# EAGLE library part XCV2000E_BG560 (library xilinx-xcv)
xcv2000e_bg560 edit this description Auto generated by make-symbol-device-package-bsdl.ulp Rev. 26 Source: xcv2000e_bg560.bsd
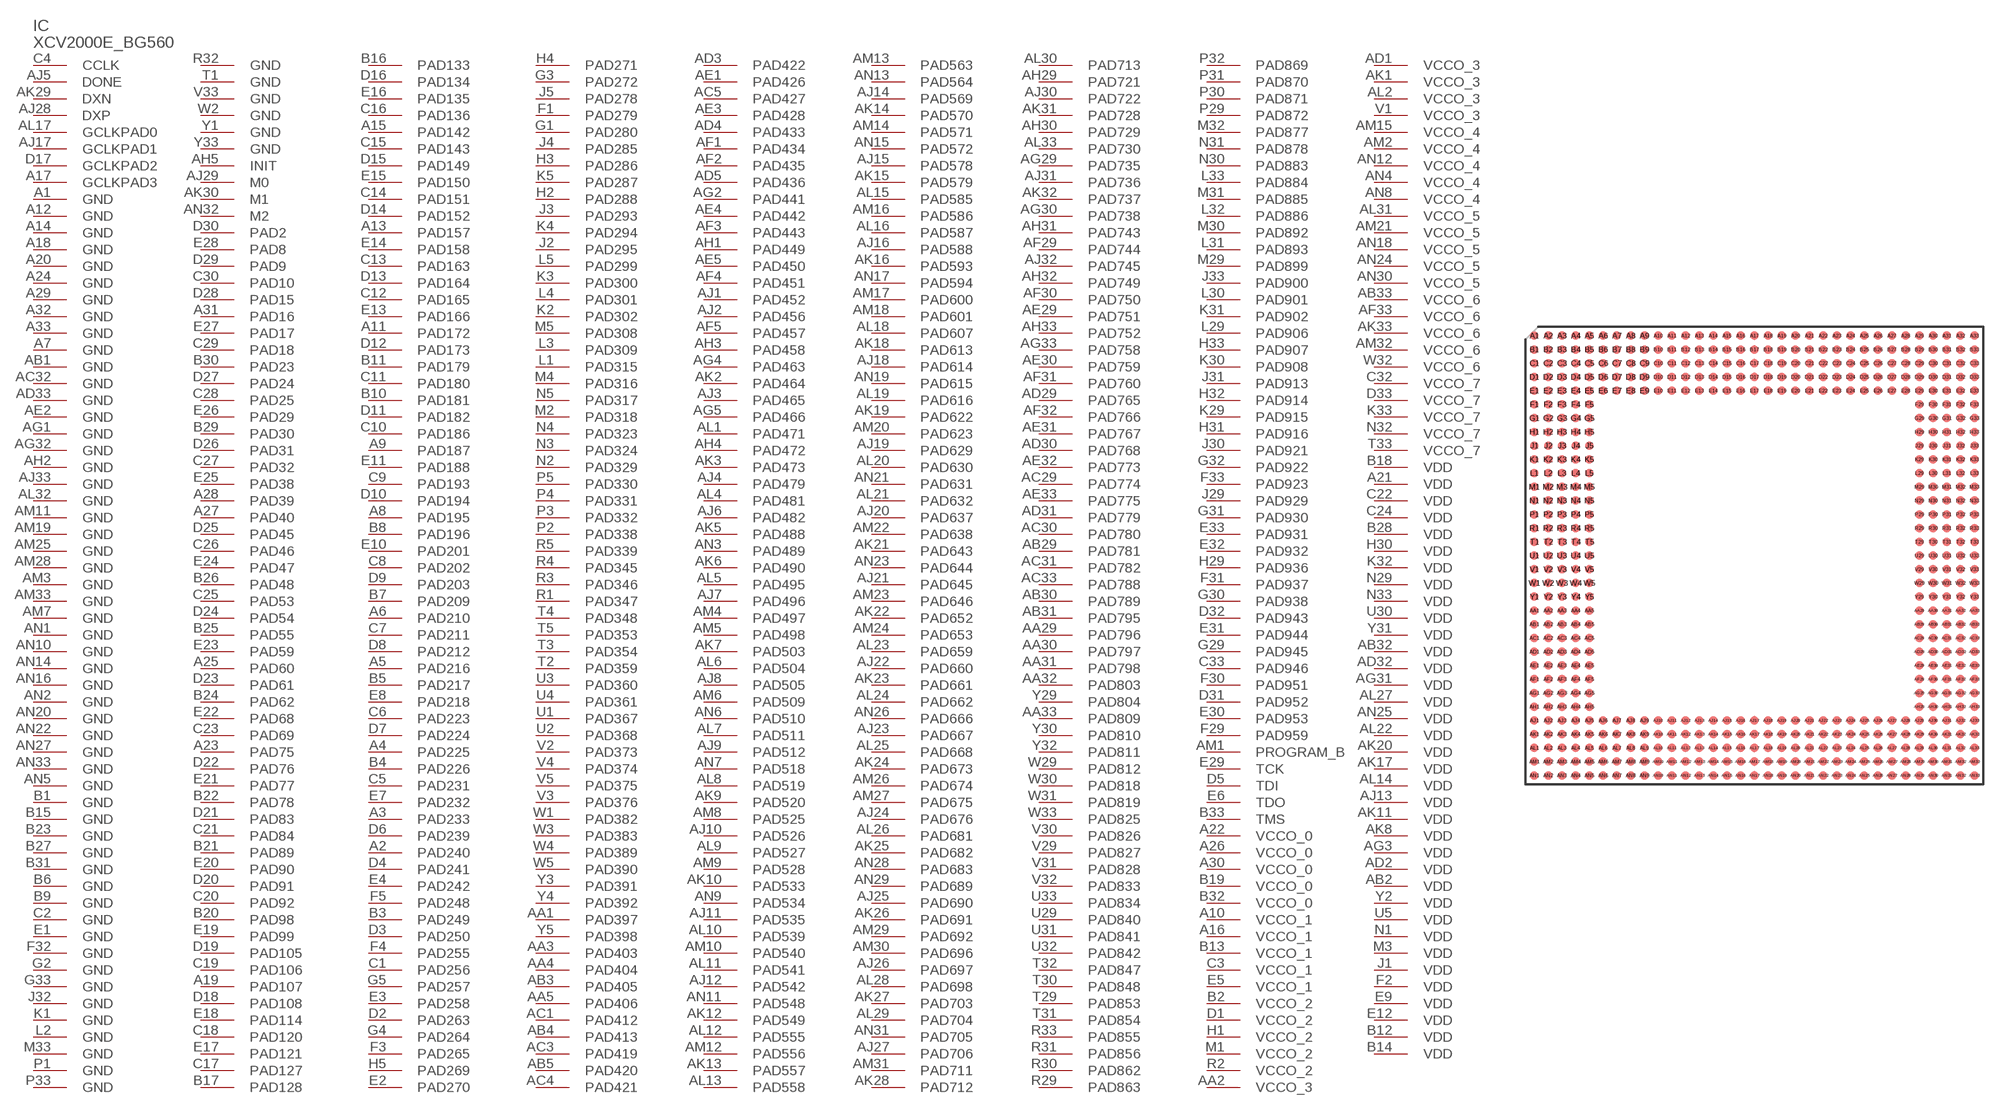
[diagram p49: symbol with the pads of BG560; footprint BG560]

Designator prefix IC

## XCV2000E_BG560 (OC_FARNELL: unknown; OC_NEWARK: unknown)  [BG560]
A1  GND  pwr
A2  PAD240
A3  PAD233
A4  PAD225
A5  PAD216
A6  PAD210
A7  GND  pwr
A8  PAD195
A9  PAD187
A10  VCCO_1  pwr
A11  PAD172
A12  GND  pwr
A13  PAD157
A14  GND  pwr
A15  PAD142
A16  VCCO_1  pwr
A17  GCLKPAD3  in
A18  GND  pwr
A19  PAD107
A20  GND  pwr
A21  VDD  pwr
A22  VCCO_0  pwr
A23  PAD75
A24  GND  pwr
A25  PAD60
A26  VCCO_0  pwr
A27  PAD40
A28  PAD39
A29  GND  pwr
A30  VCCO_0  pwr
A31  PAD16
A32  GND  pwr
A33  GND  pwr
AA1  PAD397
AA2  VCCO_3  pwr
AA3  PAD403
AA4  PAD404
AA5  PAD406
AA29  PAD796
AA30  PAD797
AA31  PAD798
AA32  PAD803
AA33  PAD809
AB1  GND  pwr
AB2  VDD  pwr
AB3  PAD405
AB4  PAD413
AB5  PAD420
AB29  PAD781
AB30  PAD789
AB31  PAD795
AB32  VDD  pwr
AB33  VCCO_6  pwr
AC1  PAD412
AC3  PAD419
AC4  PAD421
AC5  PAD427
AC29  PAD774
AC30  PAD780
AC31  PAD782
AC32  GND  pwr
AC33  PAD788
AD1  VCCO_3  pwr
AD2  VDD  pwr
AD3  PAD422
AD4  PAD433
AD5  PAD436
AD29  PAD765
AD30  PAD768
AD31  PAD779
AD32  VDD  pwr
AD33  GND  pwr
AE1  PAD426
AE2  GND  pwr
AE3  PAD428
AE4  PAD442
AE5  PAD450
AE29  PAD751
AE30  PAD759
AE31  PAD767
AE32  PAD773
AE33  PAD775
AF1  PAD434
AF2  PAD435
AF3  PAD443
AF4  PAD451
AF5  PAD457
AF29  PAD744
AF30  PAD750
AF31  PAD760
AF32  PAD766
AF33  VCCO_6  pwr
AG1  GND  pwr
AG2  PAD441
AG3  VDD  pwr
AG4  PAD463
AG5  PAD466
AG29  PAD735
AG30  PAD738
AG31  VDD  pwr
AG32  GND  pwr
AG33  PAD758
AH1  PAD449
AH2  GND  pwr
AH3  PAD458
AH4  PAD472
AH5  INIT
AH29  PAD721
AH30  PAD729
AH31  PAD743
AH32  PAD749
AH33  PAD752
AJ1  PAD452
AJ2  PAD456
AJ3  PAD465
AJ4  PAD479
AJ5  DONE
AJ6  PAD482
AJ7  PAD496
AJ8  PAD505
AJ9  PAD512
AJ10  PAD526
AJ11  PAD535
AJ12  PAD542
AJ13  VDD  pwr
AJ14  PAD569
AJ15  PAD578
AJ16  PAD588
AJ17  GCLKPAD1  in
AJ18  PAD614
AJ19  PAD629
AJ20  PAD637
AJ21  PAD645
AJ22  PAD660
AJ23  PAD667
AJ24  PAD676
AJ25  PAD690
AJ26  PAD697
AJ27  PAD706
AJ28  DXP  pas
AJ29  M0  in
AJ30  PAD722
AJ31  PAD736
AJ32  PAD745
AJ33  GND  pwr
AK1  VCCO_3  pwr
AK2  PAD464
AK3  PAD473
AK5  PAD488
AK6  PAD490
AK7  PAD503
AK8  VDD  pwr
AK9  PAD520
AK10  PAD533
AK11  VDD  pwr
AK12  PAD549
AK13  PAD557
AK14  PAD570
AK15  PAD579
AK16  PAD593
AK17  VDD  pwr
AK18  PAD613
AK19  PAD622
AK20  VDD  pwr
AK21  PAD643
AK22  PAD652
AK23  PAD661
AK24  PAD673
AK25  PAD682
AK26  PAD691
AK27  PAD703
AK28  PAD712
AK29  DXN  pas
AK30  M1  in
AK31  PAD728
AK32  PAD737
AK33  VCCO_6  pwr
AL1  PAD471
AL2  VCCO_3  pwr
AL4  PAD481
AL5  PAD495
AL6  PAD504
AL7  PAD511
AL8  PAD519
AL9  PAD527
AL10  PAD539
AL11  PAD541
AL12  PAD555
AL13  PAD558
AL14  VDD  pwr
AL15  PAD585
AL16  PAD587
AL17  GCLKPAD0  in
AL18  PAD607
AL19  PAD616
AL20  PAD630
AL21  PAD632
AL22  VDD  pwr
AL23  PAD659
AL24  PAD662
AL25  PAD668
AL26  PAD681
AL27  VDD  pwr
AL28  PAD698
AL29  PAD704
AL30  PAD713
AL31  VCCO_5  pwr
AL32  GND  pwr
AL33  PAD730
AM1  PROGRAM_B  in
AM2  VCCO_4  pwr
AM3  GND  pwr
AM4  PAD497
AM5  PAD498
AM6  PAD509
AM7  GND  pwr
AM8  PAD525
AM9  PAD528
AM10  PAD540
AM11  GND  pwr
AM12  PAD556
AM13  PAD563
AM14  PAD571
AM15  VCCO_4  pwr
AM16  PAD586
AM17  PAD600
AM18  PAD601
AM19  GND  pwr
AM20  PAD623
AM21  VCCO_5  pwr
AM22  PAD638
AM23  PAD646
AM24  PAD653
AM25  GND  pwr
AM26  PAD674
AM27  PAD675
AM28  GND  pwr
AM29  PAD692
AM30  PAD696
AM31  PAD711
AM32  VCCO_6  pwr
AM33  GND  pwr
AN1  GND  pwr
AN2  GND  pwr
AN3  PAD489
AN4  VCCO_4  pwr
AN5  GND  pwr
AN6  PAD510
AN7  PAD518
AN8  VCCO_4  pwr
AN9  PAD534
AN10  GND  pwr
AN11  PAD548
AN12  VCCO_4  pwr
AN13  PAD564
AN14  GND  pwr
AN15  PAD572
AN16  GND  pwr
AN17  PAD594
AN18  VCCO_5  pwr
AN19  PAD615
AN20  GND  pwr
AN21  PAD631
AN22  GND  pwr
AN23  PAD644
AN24  VCCO_5  pwr
AN25  VDD  pwr
AN26  PAD666
AN27  GND  pwr
AN28  PAD683
AN29  PAD689
AN30  VCCO_5  pwr
AN31  PAD705
AN32  M2  in
AN33  GND  pwr
B1  GND  pwr
B2  VCCO_2  pwr
B3  PAD249
B4  PAD226
B5  PAD217
B6  GND  pwr
B7  PAD209
B8  PAD196
B9  GND  pwr
B10  PAD181
B11  PAD179
B12  VDD  pwr
B13  VCCO_1  pwr
B14  VDD  pwr
B15  GND  pwr
B16  PAD133
B17  PAD128
B18  VDD  pwr
B19  VCCO_0  pwr
B20  PAD98
B21  PAD89
B22  PAD78
B23  GND  pwr
B24  PAD62
B25  PAD55
B26  PAD48
B27  GND  pwr
B28  VDD  pwr
B29  PAD30
B30  PAD23
B31  GND  pwr
B32  VCCO_0  pwr
B33  TMS  in
C1  PAD256
C2  GND  pwr
C3  VCCO_1  pwr
C4  CCLK
C5  PAD231
C6  PAD223
C7  PAD211
C8  PAD202
C9  PAD193
C10  PAD186
C11  PAD180
C12  PAD165
C13  PAD163
C14  PAD151
C15  PAD143
C16  PAD136
C17  PAD127
C18  PAD120
C19  PAD106
C20  PAD92
C21  PAD84
C22  VDD  pwr
C23  PAD69
C24  VDD  pwr
C25  PAD53
C26  PAD46
C27  PAD32
C28  PAD25
C29  PAD18
C30  PAD10
C32  VCCO_7  pwr
C33  PAD946
D1  VCCO_2  pwr
D2  PAD263
D3  PAD250
D4  PAD241
D5  TDI  in
D6  PAD239
D7  PAD224
D8  PAD212
D9  PAD203
D10  PAD194
D11  PAD182
D12  PAD173
D13  PAD164
D14  PAD152
D15  PAD149
D16  PAD134
D17  GCLKPAD2  in
D18  PAD108
D19  PAD105
D20  PAD91
D21  PAD83
D22  PAD76
D23  PAD61
D24  PAD54
D25  PAD45
D26  PAD31
D27  PAD24
D28  PAD15
D29  PAD9
D30  PAD2
D31  PAD952
D32  PAD943
D33  VCCO_7  pwr
E1  GND  pwr
E2  PAD270
E3  PAD258
E4  PAD242
E5  VCCO_1  pwr
E6  TDO  out
E7  PAD232
E8  PAD218
E9  VDD  pwr
E10  PAD201
E11  PAD188
E12  VDD  pwr
E13  PAD166
E14  PAD158
E15  PAD150
E16  PAD135
E17  PAD121
E18  PAD114
E19  PAD99
E20  PAD90
E21  PAD77
E22  PAD68
E23  PAD59
E24  PAD47
E25  PAD38
E26  PAD29
E27  PAD17
E28  PAD8
E29  TCK  in
E30  PAD953
E31  PAD944
E32  PAD932
E33  PAD931
F1  PAD279
F2  VDD  pwr
F3  PAD265
F4  PAD255
F5  PAD248
F29  PAD959
F30  PAD951
F31  PAD937
F32  GND  pwr
F33  PAD923
G1  PAD280
G2  GND  pwr
G3  PAD272
G4  PAD264
G5  PAD257
G29  PAD945
G30  PAD938
G31  PAD930
G32  PAD922
G33  GND  pwr
H1  VCCO_2  pwr
H2  PAD288
H3  PAD286
H4  PAD271
H5  PAD269
H29  PAD936
H30  VDD  pwr
H31  PAD916
H32  PAD914
H33  PAD907
J1  VDD  pwr
J2  PAD295
J3  PAD293
J4  PAD285
J5  PAD278
J29  PAD929
J30  PAD921
J31  PAD913
J32  GND  pwr
J33  PAD900
K1  GND  pwr
K2  PAD302
K3  PAD300
K4  PAD294
K5  PAD287
K29  PAD915
K30  PAD908
K31  PAD902
K32  VDD  pwr
K33  VCCO_7  pwr
L1  PAD315
L2  GND  pwr
L3  PAD309
L4  PAD301
L5  PAD299
L29  PAD906
L30  PAD901
L31  PAD893
L32  PAD886
L33  PAD884
M1  VCCO_2  pwr
M2  PAD318
M3  VDD  pwr
M4  PAD316
M5  PAD308
M29  PAD899
M30  PAD892
M31  PAD885
M32  PAD877
M33  GND  pwr
N1  VDD  pwr
N2  PAD329
N3  PAD324
N4  PAD323
N5  PAD317
N29  VDD  pwr
N30  PAD883
N31  PAD878
N32  VCCO_7  pwr
N33  VDD  pwr
P1  GND  pwr
P2  PAD338
P3  PAD332
P4  PAD331
P5  PAD330
P29  PAD872
P30  PAD871
P31  PAD870
P32  PAD869
P33  GND  pwr
R1  PAD347
R2  VCCO_2  pwr
R3  PAD346
R4  PAD345
R5  PAD339
R29  PAD863
R30  PAD862
R31  PAD856
R32  GND  pwr
R33  PAD855
T1  GND  pwr
T2  PAD359
T3  PAD354
T4  PAD348
T5  PAD353
T29  PAD853
T30  PAD848
T31  PAD854
T32  PAD847
T33  VCCO_7  pwr
U1  PAD367
U2  PAD368
U3  PAD360
U4  PAD361
U5  VDD  pwr
U29  PAD840
U30  VDD  pwr
U31  PAD841
U32  PAD842
U33  PAD834
V1  VCCO_3  pwr
V2  PAD373
V3  PAD376
V4  PAD374
V5  PAD375
V29  PAD827
V30  PAD826
V31  PAD828
V32  PAD833
V33  GND  pwr
W1  PAD382
W2  GND  pwr
W3  PAD383
W4  PAD389
W5  PAD390
W29  PAD812
W30  PAD818
W31  PAD819
W32  VCCO_6  pwr
W33  PAD825
Y1  GND  pwr
Y2  VDD  pwr
Y3  PAD391
Y4  PAD392
Y5  PAD398
Y29  PAD804
Y30  PAD810
Y31  VDD  pwr
Y32  PAD811
Y33  GND  pwr

## Footprint BG560 (pad centres in mm)
Metal BGA (BG560) Auto generated by make-symbol-device-package-bsdl.ulp Rev. 26 Source: xcv1000_bg560_1532.bsd; bg560.pdf
smd 0.8 x 0.8: A1 -20.32,20.32; A2 -19.05,20.32; A3 -17.78,20.32; A4 -16.51,20.32; A5 -15.24,20.32; A6 -13.97,20.32; A7 -12.7,20.32; A8 -11.43,20.32; A9 -10.16,20.32; A10 -8.89,20.32; A11 -7.62,20.32; A12 -6.35,20.32; A13 -5.08,20.32; A14 -3.81,20.32; A15 -2.54,20.32; A16 -1.27,20.32; A17 0,20.32; A18 1.27,20.32; A19 2.54,20.32; A20 3.81,20.32; A21 5.08,20.32; A22 6.35,20.32; A23 7.62,20.32; A24 8.89,20.32; A25 10.16,20.32; A26 11.43,20.32; A27 12.7,20.32; A28 13.97,20.32; A29 15.24,20.32; A30 16.51,20.32; A31 17.78,20.32; A32 19.05,20.32; A33 20.32,20.32; AA1 -20.32,-5.08; AA2 -19.05,-5.08; AA3 -17.78,-5.08; AA4 -16.51,-5.08; AA5 -15.24,-5.08; AA29 15.24,-5.08; AA30 16.51,-5.08; AA31 17.78,-5.08; AA32 19.05,-5.08; AA33 20.32,-5.08; AB1 -20.32,-6.35; AB2 -19.05,-6.35; AB3 -17.78,-6.35; AB4 -16.51,-6.35; AB5 -15.24,-6.35; AB29 15.24,-6.35; AB30 16.51,-6.35; AB31 17.78,-6.35; AB32 19.05,-6.35; AB33 20.32,-6.35; AC1 -20.32,-7.62; AC2 -19.05,-7.62; AC3 -17.78,-7.62; AC4 -16.51,-7.62; AC5 -15.24,-7.62; AC29 15.24,-7.62; AC30 16.51,-7.62; AC31 17.78,-7.62; AC32 19.05,-7.62; AC33 20.32,-7.62; AD1 -20.32,-8.89; AD2 -19.05,-8.89; AD3 -17.78,-8.89; AD4 -16.51,-8.89; AD5 -15.24,-8.89; AD29 15.24,-8.89; AD30 16.51,-8.89; AD31 17.78,-8.89; AD32 19.05,-8.89; AD33 20.32,-8.89; AE1 -20.32,-10.16; AE2 -19.05,-10.16; AE3 -17.78,-10.16; AE4 -16.51,-10.16; AE5 -15.24,-10.16; AE29 15.24,-10.16; AE30 16.51,-10.16; AE31 17.78,-10.16; AE32 19.05,-10.16; AE33 20.32,-10.16; AF1 -20.32,-11.43; AF2 -19.05,-11.43; AF3 -17.78,-11.43; AF4 -16.51,-11.43; AF5 -15.24,-11.43; AF29 15.24,-11.43; AF30 16.51,-11.43; AF31 17.78,-11.43; AF32 19.05,-11.43; AF33 20.32,-11.43; AG1 -20.32,-12.7; AG2 -19.05,-12.7; AG3 -17.78,-12.7; AG4 -16.51,-12.7; AG5 -15.24,-12.7; AG29 15.24,-12.7; AG30 16.51,-12.7; AG31 17.78,-12.7; AG32 19.05,-12.7; AG33 20.32,-12.7; AH1 -20.32,-13.97; AH2 -19.05,-13.97; AH3 -17.78,-13.97; AH4 -16.51,-13.97; AH5 -15.24,-13.97; AH29 15.24,-13.97; AH30 16.51,-13.97; AH31 17.78,-13.97; AH32 19.05,-13.97; AH33 20.32,-13.97; AJ1 -20.32,-15.24; AJ2 -19.05,-15.24; AJ3 -17.78,-15.24; AJ4 -16.51,-15.24; AJ5 -15.24,-15.24; AJ6 -13.97,-15.24; AJ7 -12.7,-15.24; AJ8 -11.43,-15.24; AJ9 -10.16,-15.24; AJ10 -8.89,-15.24; AJ11 -7.62,-15.24; AJ12 -6.35,-15.24; AJ13 -5.08,-15.24; AJ14 -3.81,-15.24; AJ15 -2.54,-15.24; AJ16 -1.27,-15.24; AJ17 0,-15.24; AJ18 1.27,-15.24; AJ19 2.54,-15.24; AJ20 3.81,-15.24; AJ21 5.08,-15.24; AJ22 6.35,-15.24; AJ23 7.62,-15.24; AJ24 8.89,-15.24; AJ25 10.16,-15.24; AJ26 11.43,-15.24; AJ27 12.7,-15.24; AJ28 13.97,-15.24; AJ29 15.24,-15.24; AJ30 16.51,-15.24; AJ31 17.78,-15.24; AJ32 19.05,-15.24; AJ33 20.32,-15.24; AK1 -20.32,-16.51; AK2 -19.05,-16.51; AK3 -17.78,-16.51; AK4 -16.51,-16.51; AK5 -15.24,-16.51; AK6 -13.97,-16.51; AK7 -12.7,-16.51; AK8 -11.43,-16.51; AK9 -10.16,-16.51; AK10 -8.89,-16.51; AK11 -7.62,-16.51; AK12 -6.35,-16.51; AK13 -5.08,-16.51; AK14 -3.81,-16.51; AK15 -2.54,-16.51; AK16 -1.27,-16.51; AK17 0,-16.51; AK18 1.27,-16.51; AK19 2.54,-16.51; AK20 3.81,-16.51; AK21 5.08,-16.51; AK22 6.35,-16.51; AK23 7.62,-16.51; AK24 8.89,-16.51; AK25 10.16,-16.51; AK26 11.43,-16.51; AK27 12.7,-16.51; AK28 13.97,-16.51; AK29 15.24,-16.51; AK30 16.51,-16.51; AK31 17.78,-16.51; AK32 19.05,-16.51; AK33 20.32,-16.51; AL1 -20.32,-17.78; AL2 -19.05,-17.78; AL3 -17.78,-17.78; AL4 -16.51,-17.78; AL5 -15.24,-17.78; AL6 -13.97,-17.78; AL7 -12.7,-17.78; AL8 -11.43,-17.78; AL9 -10.16,-17.78; AL10 -8.89,-17.78; AL11 -7.62,-17.78; AL12 -6.35,-17.78; AL13 -5.08,-17.78; AL14 -3.81,-17.78; AL15 -2.54,-17.78; AL16 -1.27,-17.78; AL17 0,-17.78; AL18 1.27,-17.78; AL19 2.54,-17.78; AL20 3.81,-17.78; AL21 5.08,-17.78; AL22 6.35,-17.78; AL23 7.62,-17.78; AL24 8.89,-17.78; AL25 10.16,-17.78; AL26 11.43,-17.78; AL27 12.7,-17.78; AL28 13.97,-17.78; AL29 15.24,-17.78; AL30 16.51,-17.78; AL31 17.78,-17.78; AL32 19.05,-17.78; AL33 20.32,-17.78; AM1 -20.32,-19.05; AM2 -19.05,-19.05; AM3 -17.78,-19.05; AM4 -16.51,-19.05; AM5 -15.24,-19.05; AM6 -13.97,-19.05; AM7 -12.7,-19.05; AM8 -11.43,-19.05; AM9 -10.16,-19.05; AM10 -8.89,-19.05; AM11 -7.62,-19.05; AM12 -6.35,-19.05; AM13 -5.08,-19.05; AM14 -3.81,-19.05; AM15 -2.54,-19.05; AM16 -1.27,-19.05; AM17 0,-19.05; AM18 1.27,-19.05; AM19 2.54,-19.05; AM20 3.81,-19.05; AM21 5.08,-19.05; AM22 6.35,-19.05; AM23 7.62,-19.05; AM24 8.89,-19.05; AM25 10.16,-19.05; AM26 11.43,-19.05; AM27 12.7,-19.05; AM28 13.97,-19.05; AM29 15.24,-19.05; AM30 16.51,-19.05; AM31 17.78,-19.05; AM32 19.05,-19.05; AM33 20.32,-19.05; AN1 -20.32,-20.32; AN2 -19.05,-20.32; AN3 -17.78,-20.32; AN4 -16.51,-20.32; AN5 -15.24,-20.32; AN6 -13.97,-20.32; AN7 -12.7,-20.32; AN8 -11.43,-20.32; AN9 -10.16,-20.32; AN10 -8.89,-20.32; AN11 -7.62,-20.32; AN12 -6.35,-20.32; AN13 -5.08,-20.32; AN14 -3.81,-20.32; AN15 -2.54,-20.32; AN16 -1.27,-20.32; AN17 0,-20.32; AN18 1.27,-20.32; AN19 2.54,-20.32; AN20 3.81,-20.32; AN21 5.08,-20.32; AN22 6.35,-20.32; AN23 7.62,-20.32; AN24 8.89,-20.32; AN25 10.16,-20.32; AN26 11.43,-20.32; AN27 12.7,-20.32; AN28 13.97,-20.32; AN29 15.24,-20.32; AN30 16.51,-20.32; AN31 17.78,-20.32; AN32 19.05,-20.32; AN33 20.32,-20.32; B1 -20.32,19.05; B2 -19.05,19.05; B3 -17.78,19.05; B4 -16.51,19.05; B5 -15.24,19.05; B6 -13.97,19.05; B7 -12.7,19.05; B8 -11.43,19.05; B9 -10.16,19.05; B10 -8.89,19.05; B11 -7.62,19.05; B12 -6.35,19.05; B13 -5.08,19.05; B14 -3.81,19.05; B15 -2.54,19.05; B16 -1.27,19.05; B17 0,19.05; B18 1.27,19.05; B19 2.54,19.05; B20 3.81,19.05; B21 5.08,19.05; B22 6.35,19.05; B23 7.62,19.05; B24 8.89,19.05; B25 10.16,19.05; B26 11.43,19.05; B27 12.7,19.05; B28 13.97,19.05; B29 15.24,19.05; B30 16.51,19.05; B31 17.78,19.05; B32 19.05,19.05; B33 20.32,19.05; C1 -20.32,17.78; C2 -19.05,17.78; C3 -17.78,17.78; C4 -16.51,17.78; C5 -15.24,17.78; C6 -13.97,17.78; C7 -12.7,17.78; C8 -11.43,17.78; C9 -10.16,17.78; C10 -8.89,17.78; C11 -7.62,17.78; C12 -6.35,17.78; C13 -5.08,17.78; C14 -3.81,17.78; C15 -2.54,17.78; C16 -1.27,17.78; C17 0,17.78; C18 1.27,17.78; C19 2.54,17.78; C20 3.81,17.78; C21 5.08,17.78; C22 6.35,17.78; C23 7.62,17.78; C24 8.89,17.78; C25 10.16,17.78; C26 11.43,17.78; C27 12.7,17.78; C28 13.97,17.78; C29 15.24,17.78; C30 16.51,17.78; C31 17.78,17.78; C32 19.05,17.78; C33 20.32,17.78; D1 -20.32,16.51; D2 -19.05,16.51; D3 -17.78,16.51; D4 -16.51,16.51; D5 -15.24,16.51; D6 -13.97,16.51; D7 -12.7,16.51; D8 -11.43,16.51; D9 -10.16,16.51; D10 -8.89,16.51; D11 -7.62,16.51; D12 -6.35,16.51; D13 -5.08,16.51; D14 -3.81,16.51; D15 -2.54,16.51; D16 -1.27,16.51; D17 0,16.51; D18 1.27,16.51; D19 2.54,16.51; D20 3.81,16.51; D21 5.08,16.51; D22 6.35,16.51; D23 7.62,16.51; D24 8.89,16.51; D25 10.16,16.51; D26 11.43,16.51; D27 12.7,16.51; D28 13.97,16.51; D29 15.24,16.51; D30 16.51,16.51; D31 17.78,16.51; D32 19.05,16.51; D33 20.32,16.51; E1 -20.32,15.24; E2 -19.05,15.24; E3 -17.78,15.24; E4 -16.51,15.24; E5 -15.24,15.24; E6 -13.97,15.24; E7 -12.7,15.24; E8 -11.43,15.24; E9 -10.16,15.24; E10 -8.89,15.24; E11 -7.62,15.24; E12 -6.35,15.24; E13 -5.08,15.24; E14 -3.81,15.24; E15 -2.54,15.24; E16 -1.27,15.24; E17 0,15.24; E18 1.27,15.24; E19 2.54,15.24; E20 3.81,15.24; E21 5.08,15.24; E22 6.35,15.24; E23 7.62,15.24; E24 8.89,15.24; E25 10.16,15.24; E26 11.43,15.24; E27 12.7,15.24; E28 13.97,15.24; E29 15.24,15.24; E30 16.51,15.24; E31 17.78,15.24; E32 19.05,15.24; E33 20.32,15.24; F1 -20.32,13.97; F2 -19.05,13.97; F3 -17.78,13.97; F4 -16.51,13.97; F5 -15.24,13.97; F29 15.24,13.97; F30 16.51,13.97; F31 17.78,13.97; F32 19.05,13.97; F33 20.32,13.97; G1 -20.32,12.7; G2 -19.05,12.7; G3 -17.78,12.7; G4 -16.51,12.7; G5 -15.24,12.7; G29 15.24,12.7; G30 16.51,12.7; G31 17.78,12.7; G32 19.05,12.7; G33 20.32,12.7; H1 -20.32,11.43; H2 -19.05,11.43; H3 -17.78,11.43; H4 -16.51,11.43; H5 -15.24,11.43; H29 15.24,11.43; H30 16.51,11.43; H31 17.78,11.43; H32 19.05,11.43; H33 20.32,11.43; J1 -20.32,10.16; J2 -19.05,10.16; J3 -17.78,10.16; J4 -16.51,10.16; J5 -15.24,10.16; J29 15.24,10.16; J30 16.51,10.16; J31 17.78,10.16; J32 19.05,10.16; J33 20.32,10.16; K1 -20.32,8.89; K2 -19.05,8.89; K3 -17.78,8.89; K4 -16.51,8.89; K5 -15.24,8.89; K29 15.24,8.89; K30 16.51,8.89; K31 17.78,8.89; K32 19.05,8.89; K33 20.32,8.89; L1 -20.32,7.62; L2 -19.05,7.62; L3 -17.78,7.62; L4 -16.51,7.62; L5 -15.24,7.62; L29 15.24,7.62; L30 16.51,7.62; L31 17.78,7.62; L32 19.05,7.62; L33 20.32,7.62; M1 -20.32,6.35; M2 -19.05,6.35; M3 -17.78,6.35; M4 -16.51,6.35; M5 -15.24,6.35; M29 15.24,6.35; M30 16.51,6.35; M31 17.78,6.35; M32 19.05,6.35; M33 20.32,6.35; N1 -20.32,5.08; N2 -19.05,5.08; N3 -17.78,5.08; N4 -16.51,5.08; N5 -15.24,5.08; N29 15.24,5.08; N30 16.51,5.08; N31 17.78,5.08; N32 19.05,5.08; N33 20.32,5.08; P1 -20.32,3.81; P2 -19.05,3.81; P3 -17.78,3.81; P4 -16.51,3.81; P5 -15.24,3.81; P29 15.24,3.81; P30 16.51,3.81; P31 17.78,3.81; P32 19.05,3.81; P33 20.32,3.81; R1 -20.32,2.54; R2 -19.05,2.54; R3 -17.78,2.54; R4 -16.51,2.54; R5 -15.24,2.54; R29 15.24,2.54; R30 16.51,2.54; R31 17.78,2.54; R32 19.05,2.54; R33 20.32,2.54; T1 -20.32,1.27; T2 -19.05,1.27; T3 -17.78,1.27; T4 -16.51,1.27; T5 -15.24,1.27; T29 15.24,1.27; T30 16.51,1.27; T31 17.78,1.27; T32 19.05,1.27; T33 20.32,1.27; U1 -20.32,0; U2 -19.05,0; U3 -17.78,0; U4 -16.51,0; U5 -15.24,0; U29 15.24,0; U30 16.51,0; U31 17.78,0; U32 19.05,0; U33 20.32,0; V1 -20.32,-1.27; V2 -19.05,-1.27; V3 -17.78,-1.27; V4 -16.51,-1.27; V5 -15.24,-1.27; V29 15.24,-1.27; V30 16.51,-1.27; V31 17.78,-1.27; V32 19.05,-1.27; V33 20.32,-1.27; W1 -20.32,-2.54; W2 -19.05,-2.54; W3 -17.78,-2.54; W4 -16.51,-2.54; W5 -15.24,-2.54; W29 15.24,-2.54; W30 16.51,-2.54; W31 17.78,-2.54; W32 19.05,-2.54; W33 20.32,-2.54; Y1 -20.32,-3.81; Y2 -19.05,-3.81; Y3 -17.78,-3.81; Y4 -16.51,-3.81; Y5 -15.24,-3.81; Y29 15.24,-3.81; Y30 16.51,-3.81; Y31 17.78,-3.81; Y32 19.05,-3.81; Y33 20.32,-3.81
